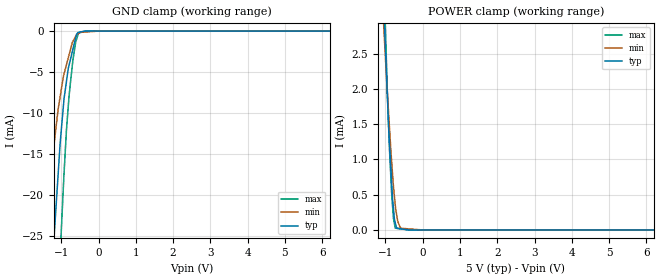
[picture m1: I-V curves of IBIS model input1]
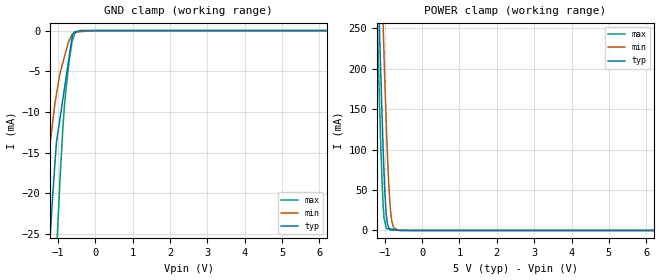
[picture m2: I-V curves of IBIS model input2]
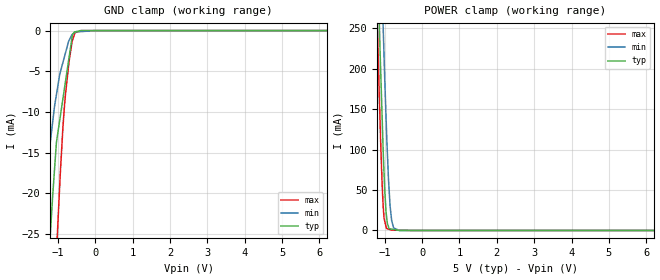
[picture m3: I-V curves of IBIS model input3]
| Texas Instruments Incorporated
|ADS125H0x Wide-Input Range, 2-Channel, 19.2-kSPS, 24-Bit, Delta-Sigma ADC
|With PGA and Voltage Reference
[IBIS Ver]   4.1
[File name]   ads125h0x.ibs
[File Rev]   1.0
[Date]   04/13/2018
[Source]
| Texas Instruments Incorporated.
| Analog-eLab Design Center, HPA
| 12500 TI Blvd
| Dallas, TX -75243
[Notes]   Revision History:
| Rev 1.0: 04/13/2018
| - Initial version of the model
| - Model generated from simulations in SPECTRE
| - C_comp although listed in numerical order of value are
|   obtained from varying PVT conditions. For PVT conditions for
|   each specific value refer the buffer description under
|   respective [Model]. IBIS model user is responsible for using
|   appropriate C_comp to simulate for Signal Integrity.
| - Warnings regarding combined Non-monotonicity of various models
|   have been reviewed and considered minor and can be ignored.
[Disclaimer]
| This model is designed as an aid for customers of Texas Instruments.
| TI and its licensors and suppliers make no warranties, either expressed
| or implied, with respect to this  model, including the warranties of
| merchantability or fitness for a particular purpose. The model is
| provided solely on an "as is" basis. The entire risk as to its quality
| and performance is with the customer.
| This model is subject to change without notice. Texas Instruments
| Incorporated is not responsible for updating this model.
[Copyright]
 (C) Copyright 2018 Texas Instruments Incorporated. All rights reserved.
|  Component ADS125H01 32-pin VQFN - RHB Package
|  Part # ADS125H01RHB
[Component]   ADS125H01RHB
[Manufacturer]   TI
[Package]   |32 VQFN - RHB package
|   typ   min   max
R_pkg   0.05   0.04   0.06
L_pkg   1.0nH   0.8nH   1.2nH
C_pkg   0.2pF   0.16pF   0.24pF
[Pin]   signal_name   model_name   R_pin   L_pin   C_pin
1   REFP0   nc   NA   NA   NA
2   CAPP   nc   NA   NA   NA
3   CAPN   nc   NA   NA   NA
4   AVDD   power   NA   NA   NA
5   AGND   gnd   NA   NA   NA
6   REFOUT   nc   NA   NA   NA
7   _RESET   input1   NA   NA   NA
8   START   input2   NA   NA   NA
9   _CS2   input3   NA   NA   NA
10   _CS1   input4   NA   NA   NA
11   SCLK   input4   NA   NA   NA
12   DIN   input4   NA   NA   NA
13   _DRDY   output1   NA   NA   NA
14   DOUT/_DRDY   dout   NA   NA   NA
15   BYPASS   nc   NA   NA   NA
16   DGND   gnd   NA   NA   NA
17   DVDD   power   NA   NA   NA
18   CLKIN   input5   NA   NA   NA
19   HV_AVSS   gnd   NA   NA   NA
20   HV_AVDD   power   NA   NA   NA
21   NC   nc   NA   NA   NA
22   NC   nc   NA   NA   NA
23   NC   nc   NA   NA   NA
24   NC   nc   NA   NA   NA
25   AINCOM   nc   NA   NA   NA
26   AIN0   nc   NA   NA   NA
27   AIN1   nc   NA   NA   NA
28   NC   nc   NA   NA   NA
29   NC   nc   NA   NA   NA
30   NC   nc   NA   NA   NA
31   NC   nc   NA   NA   NA
32   REFN0   nc   NA   NA   NA
|  Component ADS125H02 32-pin VQFN - RHB Package
|  Part # ADS125H02RHB
[Component]   ADS125H02RHB
[Manufacturer]   TI
[Package]   |32 VQFN - RHB package
|   typ   min   max
R_pkg   0.05   0.04   0.06
L_pkg   1.0nH   0.8nH   1.2nH
C_pkg   0.2pF   0.16pF   0.24pF
[Pin]   signal_name   model_name   R_pin   L_pin   C_pin
1   REFP0   nc   NA   NA   NA
2   CAPP   nc   NA   NA   NA
3   CAPN   nc   NA   NA   NA
4   AVDD   power   NA   NA   NA
5   AGND   gnd   NA   NA   NA
6   REFOUT   nc   NA   NA   NA
7   _RESET   input1   NA   NA   NA
8   START   input2   NA   NA   NA
9   _CS2   input3   NA   NA   NA
10   _CS1   input4   NA   NA   NA
11   SCLK   input4   NA   NA   NA
12   DIN   input4   NA   NA   NA
13   _DRDY   output1   NA   NA   NA
14   DOUT/_DRDY   dout   NA   NA   NA
15   BYPASS   nc   NA   NA   NA
16   DGND   gnd   NA   NA   NA
17   DVDD   power   NA   NA   NA
18   CLKIN   input5   NA   NA   NA
19   HV_AVSS   gnd   NA   NA   NA
20   HV_AVDD   power   NA   NA   NA
21   NC   nc   NA   NA   NA
22   NC   nc   NA   NA   NA
23   IDAC2   nc   NA   NA   NA
24   IDAC1   nc   NA   NA   NA
25   AINCOM   nc   NA   NA   NA
26   AIN0   nc   NA   NA   NA
27   AIN1   nc   NA   NA   NA
28   GPIO3   io   NA   NA   NA
29   GPIO2   io   NA   NA   NA
30   REFN1/GPIO1   io   NA   NA   NA
31   REFP1/GPIO0   io   NA   NA   NA
32   REFN0   nc   NA   NA   NA
[Model Selector] dout
dout_apache   5V   digital Output
dout_spark   5V   digital Output
| Models and submodels in the file (9): input1 (Input), input2 (Input), input3 (Input), input4 (Input), input5 (Input), io (I/O), output1 (Output), dout_apache (3-state), dout_spark (3-state)
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|   input1 Model
[Model]   input1
Model_type   Input
Vinl = 1.5
Vinh = 3.5
|   typ   min   max
C_comp   2.097pF   1.769pF   2.332pF
|  Where Nom  PVT is Nominal Process,   5V,  27C
|   Fast PVT is Strong Process,   5.25V, -40C
|   Slow PVT is Weak Process,   2.7V, 135C
[Model spec]
|subparameter
Vinl   1.500   0.810   1.575
Vinh   3.500   1.890   3.675
[Voltage Range]   5   2.7   5.25
|Junction Temperature
[Temperature Range]   27   135   -40
[Power Clamp Reference]   5   2.7   5.25
[GND Clamp Reference]   0   0   0
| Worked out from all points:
|   GND clamp passes 1 mA (typ) near -0.62 V on its own axis
|   POWER clamp passes 1 mA (typ) near -0.87 V on its own axis
[GND Clamp]
|   Voltage   I(typ)   I(min)   I(max)
-5V       -411.9mA   -286.8mA   -505.9mA
-1.431V   -44.29mA   -24.6mA    -72.55mA
-1.25V    -29.13mA   -15.99mA   -51.34mA
-1.125V   -20.36mA   -11.14mA   -37.39mA
-1.02V    -13.12mA   -7.699mA   -26.27mA
-925.5mV  -8.237mA   -5.215mA   -17.34mA
-859.4mV  -6.098mA   -4.079mA   -11.96mA
-791mV    -4.157mA   -2.903mA   -7.903mA
-691.6mV  -2.279mA   -1.289mA   -3.661mA
-613mV    -793.6uA   -632.4uA   -1.318mA
-552.1mV  -174.7uA   -320.7uA   -465.3uA
10V       0A         0A         0A
[POWER Clamp]
|   Voltage   I(typ)   I(min)   I(max)
-5V       83.73mA    65.22mA    101.9mA
-1.066V   3.562mA    3.079mA    4.189mA
-1.03V    2.953mA    2.734mA    3.452mA
-1.003V   2.596mA    2.462mA    2.902mA
-895.1mV  1.272mA    1.477mA    1.176mA
-834.1mV  673.8uA    972.1uA    517.1uA
-785.2mV  299.6uA    615.8uA    163.3uA
-736.6mV  99.9uA     351.5uA    25.61uA
-671.1mV  23.45uA    123.9uA    21uA
-592.2mV  17.25uA    24.58uA    15.44uA
-136uV    0A         0A         0A
10V       0A         0A         0A
|   input2 Model
[Model]   input2
Model_type   Input
Vinl = 1.5
Vinh = 3.5
|   typ   min   max
C_comp   2.031pF   1.769pF   2.237pF
|  Where Nom  PVT is Nominal Process,   5V,  27C
|   Fast PVT is Strong Process,   5.25V, -40C
|   Slow PVT is Weak Process,   2.7V, 135C
[Model spec]
|subparameter
Vinl   1.500   0.810   1.575
Vinh   3.500   1.890   3.675
[Voltage Range]   5   2.7   5.25
|Junction Temperature
[Temperature Range]   27   135   -40
[Power Clamp Reference]   5   2.7   5.25
[GND Clamp Reference]   0   0   0
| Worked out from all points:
|   GND clamp passes 1 mA (typ) near -0.62 V on its own axis
|   POWER clamp passes 1 mA (typ) near -0.73 V on its own axis
[GND Clamp]
|   Voltage   I(typ)   I(min)   I(max)
-5V       -410mA     -285.3mA   -503.9mA
-1.44V    -44.59mA   -24.64mA   -73.15mA
-1.25V    -28.81mA   -15.66mA   -50.96mA
-1.136V   -20.34mA   -11.26mA   -38.24mA
-1.021V   -13.29mA   -7.467mA   -26.02mA
-861.5mV  -8.371mA   -3.915mA   -11.87mA
-793.7mV  -6.276mA   -2.755mA   -7.859mA
-694.3mV  -3.203mA   -1.183mA   -3.67mA
-607.1mV  -510.3uA   -447uA     -1.215mA
-553.2mV  -173.2uA   -262uA     -464.5uA
-368.8mV  -2.276uA   -122.5uA   -967.2nA
10V       0A         0A         0A
[POWER Clamp]
|   Voltage   I(typ)   I(min)   I(max)
-5V       7.793A     7.929A     7.725A
-1.25V    441.2mA    609.4mA    349.1mA
-1.15V    269.3mA    433.6mA    177.9mA
-1.14V    252.9mA    417.7mA    161.7mA
-1.067V   141.2mA    296mA      58.5mA
-1.036V   94.04mA    246.8mA    28.32mA
-962.5mV  23.07mA    140.7mA    4.923mA
-896.4mV  4.471mA    63.13mA    1.697mA
-821.5mV  1.806mA    16.35mA    431.7uA
-757.8mV  1.269mA    3.093mA    388.9uA
-607.2mV  1.677uA    49.97uA    287.8uA
10V       0A         0A         0A
|   input3 Model
[Model]   input3
Model_type   Input
Vinl = 1.5
Vinh = 3.5
|   typ   min   max
C_comp   2.03068pF   1.76864pF   2.23686pF
|  Where Nom  PVT is Nominal Process,   5V,  27C
|   Fast PVT is Strong Process,   5.25V, -40C
|   Slow PVT is Weak Process,   2.7V, 135C
[Model spec]
|subparameter
Vinl   1.500   0.810   1.575
Vinh   3.500   1.890   3.675
[Voltage Range]   5   2.7   5.25
|Junction Temperature
[Temperature Range]   27   135   -40
[Power Clamp Reference]   5   2.7   5.25
[GND Clamp Reference]   0   0   0
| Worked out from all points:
|   GND clamp passes 1 mA (typ) near -0.62 V on its own axis
|   POWER clamp passes 1 mA (typ) near -0.73 V on its own axis
[GND Clamp]
|   Voltage   I(typ)   I(min)   I(max)
-5V       -410mA     -285.3mA   -503.9mA
-1.44V    -44.59mA   -24.64mA   -73.15mA
-1.25V    -28.81mA   -15.66mA   -50.96mA
-1.136V   -20.34mA   -11.26mA   -38.24mA
-1.021V   -13.29mA   -7.467mA   -26.02mA
-861.5mV  -8.371mA   -3.915mA   -11.87mA
-793.7mV  -6.276mA   -2.755mA   -7.859mA
-694.3mV  -3.203mA   -1.183mA   -3.67mA
-607.1mV  -510.3uA   -447uA     -1.215mA
-553.2mV  -173.2uA   -262uA     -464.5uA
-368.8mV  -2.276uA   -122.5uA   -967.2nA
10V       0A         0A         0A
[POWER Clamp]
|   Voltage   I(typ)   I(min)   I(max)
-5V       7.793A     7.929A     7.725A
-1.25V    441.2mA    609.4mA    349.1mA
-1.15V    269.3mA    433.6mA    177.9mA
-1.14V    252.9mA    417.7mA    161.7mA
-1.067V   141.2mA    296mA      58.5mA
-1.036V   94.04mA    246.8mA    28.32mA
-962.5mV  23.07mA    140.7mA    4.923mA
-896.4mV  4.471mA    63.13mA    1.697mA
-821.5mV  1.806mA    16.35mA    431.7uA
-757.8mV  1.269mA    3.093mA    388.9uA
-607.2mV  1.677uA    49.97uA    287.8uA
10V       0A         0A         0A
